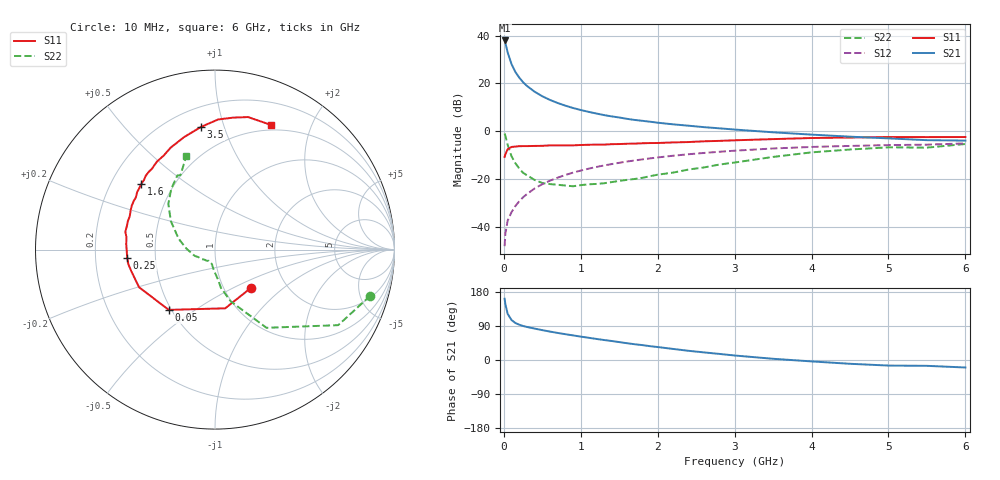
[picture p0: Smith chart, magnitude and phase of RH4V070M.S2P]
! SIEMENS Small Signal Semiconductors
! BFR106
! Si NPN RF Bipolar Junction Transistor in SOT23
! VCE = 4 V  IC = 70 mA
! Common Emitter S-Parameters:  August  1996
# GHz  S  MA  R  50
!  f  S11  S21  S12  S22
! GHz  MAG  ANG  MAG  ANG  MAG  ANG  MAG  ANG
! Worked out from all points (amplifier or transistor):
!   36 points, 10 MHz to 6 GHz, reference 50 ohm
!   highest |S21| = 38.0 dB at 10 MHz (marker M1)
!   |S21| within 3 dB of that: start of sweep to 34.62 MHz
!   unconditionally stable (mu >= 1): 212.2 MHz to 2.433 GHz
!   at 250 MHz: K = 1.03, MAG = 23.0 dB, |S12| = -27.5 dB
!   at 1.4 GHz: K = 1.06, MAG = 8.5 dB, |S12| = -13.7 dB
!   at 6 GHz: K = 0.99, MSG = 0.6 dB, |S12| = -5.0 dB
!   S11 on the Smith chart (normalised r, x): 10 MHz: 1.34, -0.62; 50 MHz: 0.48, -0.40; 250 MHz: 0.34, -0.04; 1.6 GHz: 0.33, +0.35; 3.5 GHz: 0.32, +0.84; 6 GHz: 0.44, +1.45
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0.01  0.2927 -46.6  79.05 161.6  0.004 80.3  0.9021 -16.6
0.02  0.3321 -80.1  69.96 147.1  0.0074 71.6  0.8055 -31.5
0.05  0.4233 -127.5  44.25 121.7  0.0137 61.7  0.5219 -56.6
0.1  0.4721 -153.6  25.34 105.4  0.0205 63.1  0.3024 -73.0
0.15  0.4806 -164.9  17.36 97.6  0.0275 66.9  0.2155 -81.2
0.2  0.4897 -170.5  13.25 93.2  0.0347 70.4  0.1679 -84.2
0.25  0.4911 -174.8  10.61 89.7  0.042 71.0  0.1364 -88.8
0.3  0.4916 -178.2  8.89 87.2  0.049 72.5  0.1211 -92.1
0.4  0.4956 176.4  6.722 82.9  0.0641 73.4  0.0966 -97.6
0.5  0.498 172.1  5.4 78.8  0.0787 72.8  0.0835 -101.6
0.6  0.5091 168.8  4.527 75.0  0.0933 72.3  0.0792 -105.7
0.7  0.5084 164.8  3.906 71.4  0.1079 71.3  0.0766 -110.7
0.9  0.5098 158.7  3.072 64.9  0.1375 68.6  0.0713 -119.7
1.1  0.5244 152.1  2.556 58.7  0.1658 66.0  0.0784 -128.8
1.3  0.5281 146.6  2.188 52.8  0.1936 63.1  0.0823 -137.5
1.6  0.5506 138.2  1.825 44.3  0.2339 58.6  0.097 -150.4
2.2  0.5871 123.5  1.401 29.2  0.3093 49.3  0.1375 -173.9
2.8  0.6318 109.7  1.157 16.1  0.3745 39.8  0.2022 165.3
3.5  0.6881 96.5  0.955 3.2  0.4387 29.2  0.2924 147.2
4.5  0.7427 82.0  0.774 -10.0  0.496 14.7  0.4174 125.7
5.5  0.7584 70.0  0.654 -15.4  0.5272 5.3  0.457 114.9
6  0.7611 65.9  0.641 -19.8  0.5604 -1.8  0.5444 107.1
